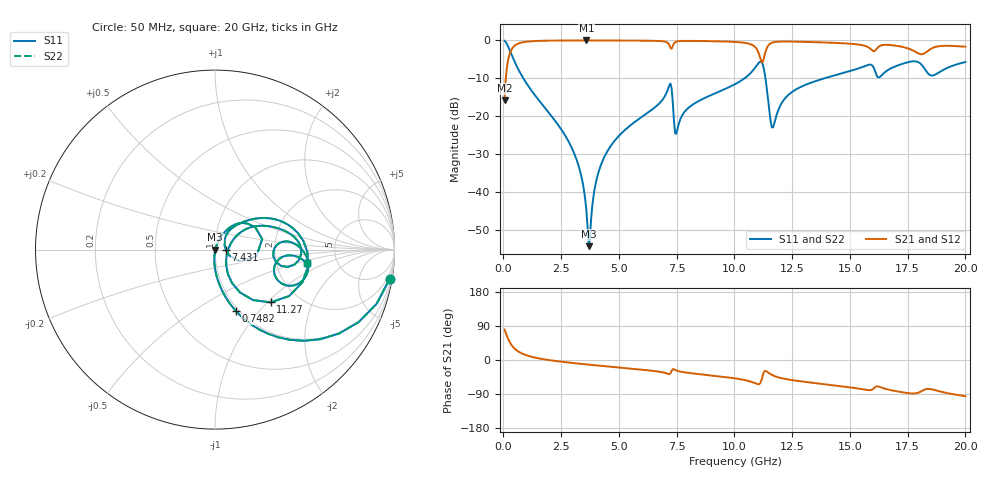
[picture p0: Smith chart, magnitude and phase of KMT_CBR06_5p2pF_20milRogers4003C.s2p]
! Data measured by Modelithics Inc. support@modelithics.com 813-866-6335
! KEMET CBR0603 5.2pF, Pad Width= 0.851mm, Pad Length= 0.64mm, Pad Gap= 0.62mm, 20mil Rogers 4003C substrate Data, January 2022
# hz S ma R 50
! 2 Port Network Data from SP1.SP block
! freq  magS11  angS11  magS21  angS21  magS12  angS12  magS22  angS22
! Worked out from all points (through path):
!   401 points, 50 MHz to 20 GHz, reference 50 ohm
!   highest |S21| = -0.02 dB at 3.591 GHz (marker M1); lowest = -15.8 dB at 50 MHz (marker M2)
!   group delay of S21, straight-line fit = 15.3 ps
!   lowest |S11| = -54.1 dB at 3.691 GHz (marker M3), VSWR 1.00, Z = 50.2 - j0.113 ohm
!   |S11| at or under -10 dB: 863.1 MHz to 10.43 GHz (9.571 GHz wide, 169 % of centre); 11.34 GHz to 13.89 GHz (2.542 GHz wide, 20.2 % of centre)
!   |S22| runs from -54.1 to -0.1 dB; largest |S21 - S12| = 0
!   S11 on the Smith chart (normalised r, x): 50 MHz: 1, -12; 748.2 MHz: 0.97, -0.77; 7.431 GHz: 1.13, -0.00; 11.27 GHz: 1.45, -1.05; 20 GHz: 3.01, -0.63
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5e7  0.9867 -9.5  0.1625 80.5  0.1625 80.5  0.9867 -9.5
2.99375e8  0.7095 -45.8  0.704 44.2  0.704 44.2  0.7095 -45.8
7.4825e8  0.363 -71.1  0.9308 18.8  0.9308 18.8  0.363 -71.1
2.74325e9  0.05143 -94.5  0.997 -6.2  0.997 -6.2  0.05143 -94.5
3.391625e9  0.01534 -94.0  0.998 -10.5  0.998 -10.5  0.01534 -94.0
3.591125e9  0.005754 -83.6  0.9981 -11.7  0.9981 -11.7  0.005754 -83.6
3.690875e9  0.001962 -34.9  0.9981 -12.3  0.9981 -12.3  0.001962 -34.9
4.04e9  0.01518 68.4  0.9978 -14.3  0.9978 -14.3  0.01518 68.4
4.488875e9  0.03433 69.7  0.9972 -16.9  0.9972 -16.9  0.03433 69.7
6.73325e9  0.1466 56.4  0.9819 -30.8  0.9819 -30.8  0.1466 56.4
7.182125e9  0.2565 28.9  0.8688 -37.4  0.8688 -37.4  0.2565 28.9
7.4315e9  0.05995 -0.6  0.9453 -26.1  0.9453 -26.1  0.05995 -0.6
1.0025e10  0.2654 39.5  0.9541 -48.5  0.9541 -48.5  0.2654 39.5
1.087288e10  0.4284 19.1  0.8305 -60.7  0.8305 -60.7  0.4284 19.1
1.127188e10  0.4275 -43.4  0.5767 -32.4  0.5767 -32.4  0.4275 -43.4
1.167088e10  0.07172 -4.2  0.9411 -40.8  0.9411 -40.8  0.07172 -4.2
1.226938e10  0.1835 34.0  0.9661 -50.8  0.9661 -50.8  0.1835 34.0
1.336662e10  0.2812 28.1  0.9502 -60.0  0.9502 -60.0  0.2812 28.1
1.670825e10  0.4181 6.0  0.87 -78.8  0.87 -78.8  0.4181 6.0
1.810475e10  0.478 -24.8  0.6569 -82.2  0.6569 -82.2  0.478 -24.8
1.855362e10  0.3445 -15.6  0.7896 -77.5  0.7896 -77.5  0.3445 -15.6
2e10  0.5194 -8.5  0.8266 -95.5  0.8266 -95.5  0.5194 -8.5
